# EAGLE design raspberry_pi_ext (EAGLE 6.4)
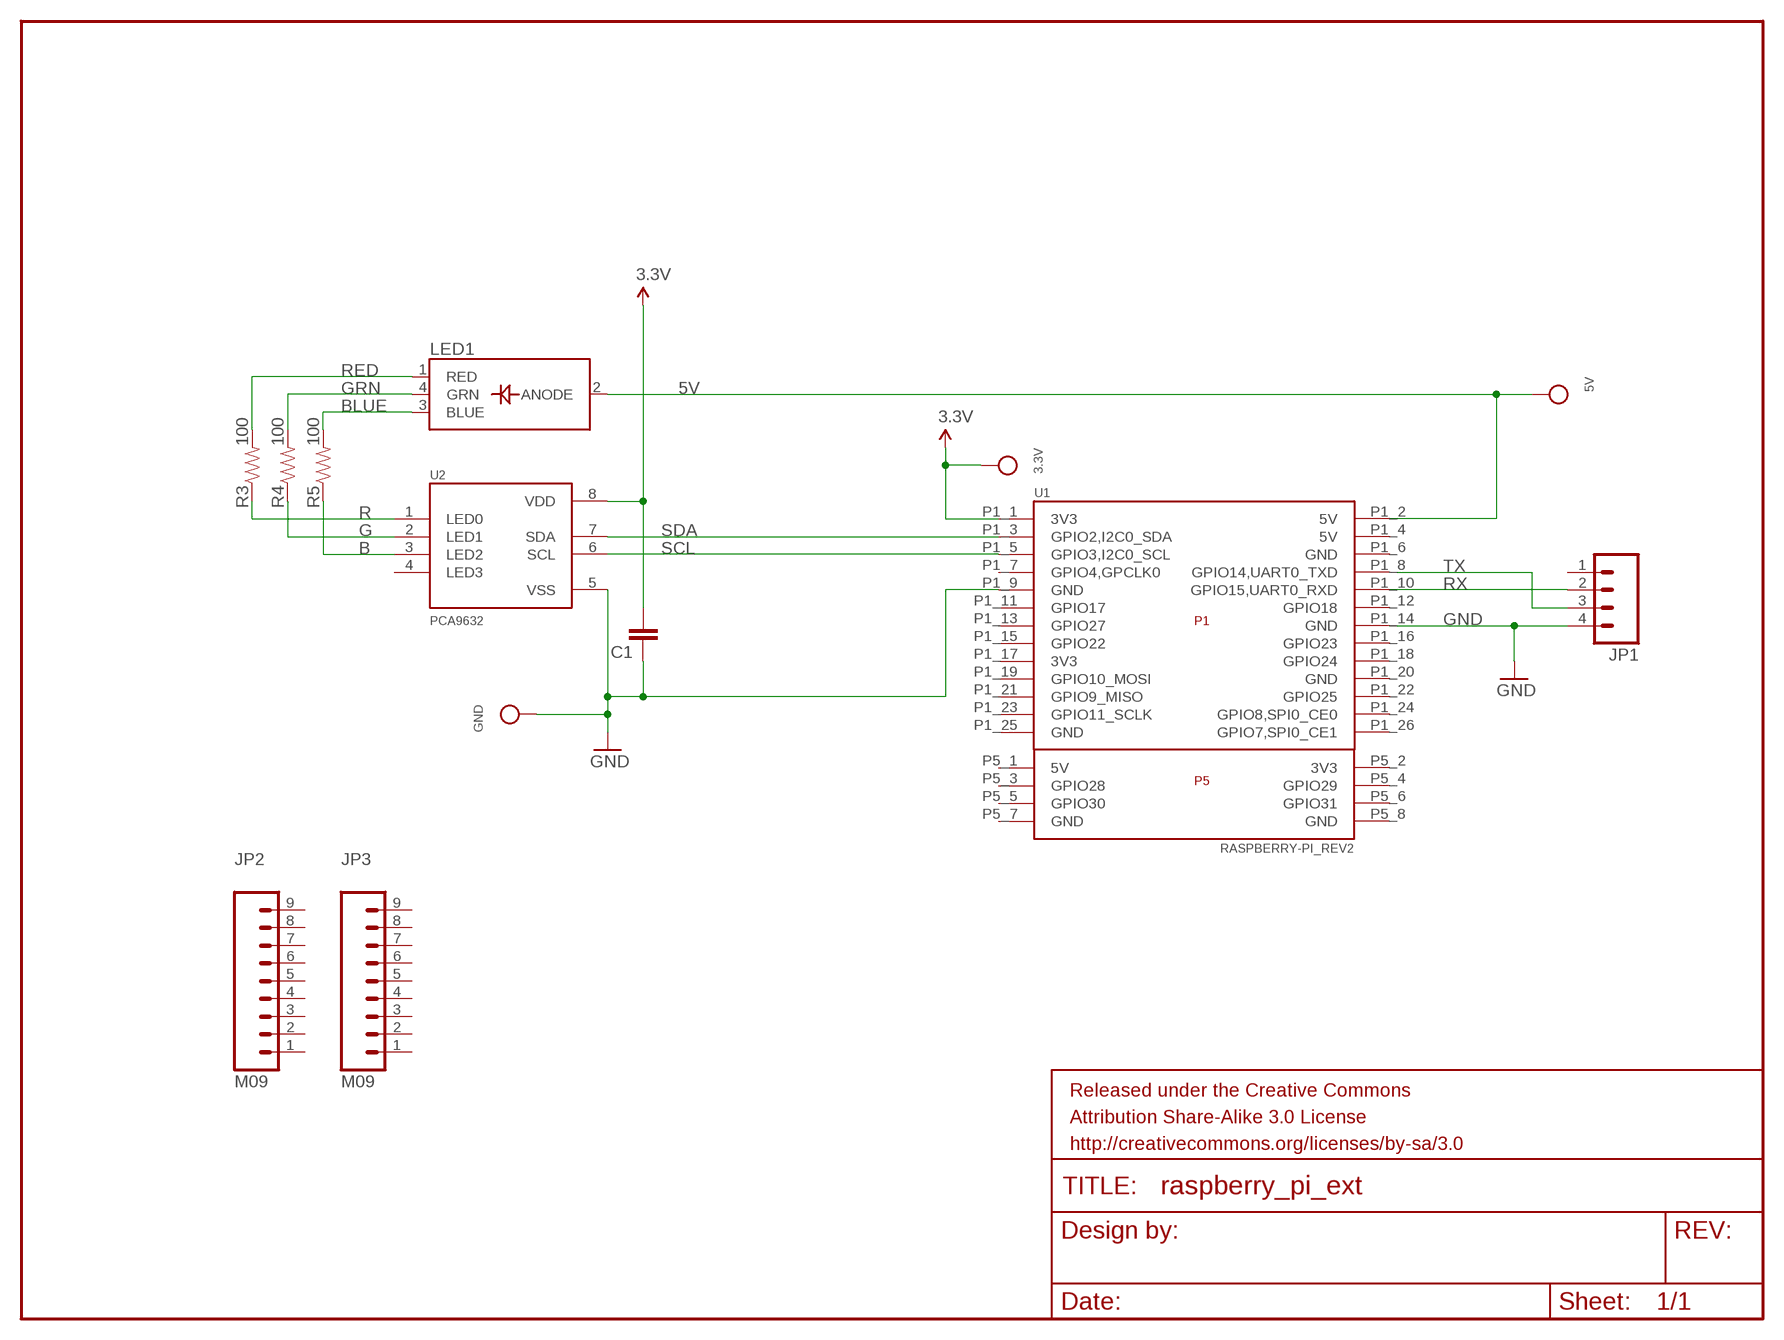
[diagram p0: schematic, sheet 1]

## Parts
3.3V  TESTPOINT0.1"  [1X01_ROUND]
5V  TESTPOINT0.1"  [1X01_ROUND]
C1  CAP0603-CAP  [0603-CAP]
FRAME1  FRAME-LETTER  [CREATIVE_COMMONS]
GND  TESTPOINT0.1"  [1X01_ROUND]
JP1  M04PTH  [1X04]
JP2  M09  [1X09]
JP3  M09  [1X09]
LED1  LED_RGB_PLCC4  [RGBLED_PLCC4]
R3  100  RESISTOR0603-RES  [0603-RES]
R4  100  RESISTOR0603-RES  [0603-RES]
R5  100  RESISTOR0603-RES  [0603-RES]
U1  RASPBERRY-PI_REV2  [RASPBERRY-PI_REV2]
U2  PCA9632  [TSSOP-8]

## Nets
3.3V: 3.3V.1 C1.2 U1.P1_1(3V3) U2.8(VDD)
5V: 5V.1 LED1.2(ANODE) U1.P1_2(5V)
B: R5.1 U2.3(LED2)
BLUE: LED1.3(BLUE) R5.2
G: R4.1 U2.2(LED1)
GND: C1.1 GND.1 JP1.4 U1.P1_9(GND) U1.P1_14(GND) U2.5(VSS)
GRN: LED1.4(GRN) R4.2
R: R3.1 U2.1(LED0)
RED: LED1.1(RED) R3.2
RX: JP1.2 U1.P1_10(GPIO15,UART0_RXD)
SCL: U1.P1_5(GPIO3,I2C0_SCL) U2.6(SCL)
SDA: U1.P1_3(GPIO2,I2C0_SDA) U2.7(SDA)
TX: JP1.3 U1.P1_8(GPIO14,UART0_TXD)
Unconnected: JP1.1 JP2.1 JP2.2 JP2.3 JP2.4 JP2.5 JP2.6 JP2.7 JP2.8 JP2.9 JP3.1 JP3.2 JP3.3 JP3.4 JP3.5 JP3.6 JP3.7 JP3.8 JP3.9 U1.P1_4(5V) U1.P1_6(GND) U1.P1_7(GPIO4,GPCLK0) U1.P1_11(GPIO17) U1.P1_12(GPIO18) U1.P1_13(GPIO27) U1.P1_15(GPIO22) U1.P1_16(GPIO23) U1.P1_17(3V3) U1.P1_18(GPIO24) U1.P1_19(GPIO10_MOSI) U1.P1_20(GND) U1.P1_21(GPIO9_MISO) U1.P1_22(GPIO25) U1.P1_23(GPIO11_SCLK) U1.P1_24(GPIO8,SPI0_CE0) U1.P1_25(GND) U1.P1_26(GPIO7,SPI0_CE1) U1.P5_1(5V) U1.P5_2(3V3) U1.P5_3(GPIO28) U1.P5_4(GPIO29) U1.P5_5(GPIO30) U1.P5_6(GPIO31) U1.P5_7(GND) U1.P5_8(GND) U2.4(LED3)

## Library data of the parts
3.3V 5V GND = microbuilder:TESTPOINT: Test Point; BOM: EXCLUDE
C1 = SparkFun-Capacitors:CAP: Capacitor
FRAME1 = SparkFun-Aesthetics:FRAME-LETTER: Schematic Frame
JP1 = SparkFun-Connectors:M04: Header 4 Standard 4-pin 0.1" header. Use with straight break away headers (SKU : PRT-00116), right angle break away headers (PRT-00553), swiss pins (PRT-00743), machine pins (PRT-00117), and female headers (PRT-00115). Molex polarized connector foot print use with SKU : PRT-08231 with associated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
JP2 JP3 = SparkFun-Connectors:M09: Header 9 Standard 9-pin 0.1" header. Use with straight break away headers (SKU : PRT-00116), right angle break away headers (PRT-00553), swiss pins (PRT-00743), machine pins (PRT-00117), and female headers (PRT-00115).
LED1 = microbuilder:LED_RGB_PLCC4: RGB LED - PLCC4 Cree 20mA Common Anode Digikey: CLV1A-FKB-CJ1M1F1BB7R4S3CT-ND Red: 2.6V Vf, 550mcd Green: 3.2V Vf, 850mcd Blue: 3.2V Vf, 320mcd
R3-R5 = SparkFun-Resistors:RESISTOR: Resistor
U1 = RaspberryPi:RASPBERRY-PI_REV2: Raspberry Pi Board Jacques Lagnel V1.0 (beta) 2012 Mateusz Bawaj V1.1 (beta) 2012 Board dimension: Forum 3D model The GPIO Connector (P1): http://elinux.org/RPi_Low-level_peripherals The GPIO Connector (P5): http://www.raspberrypi-spy.co.uk/2012/09/raspberry-pi-p5-header/
U2 = jetperch:PCA9632

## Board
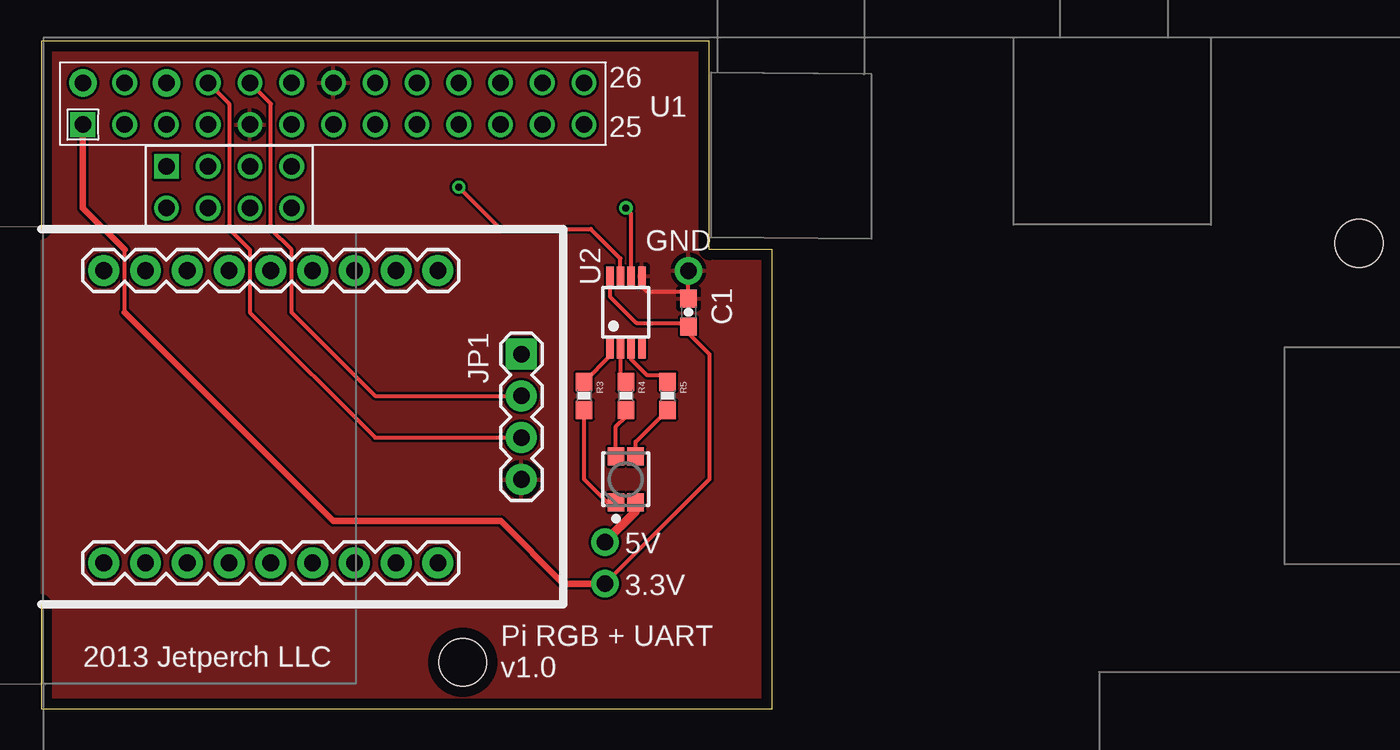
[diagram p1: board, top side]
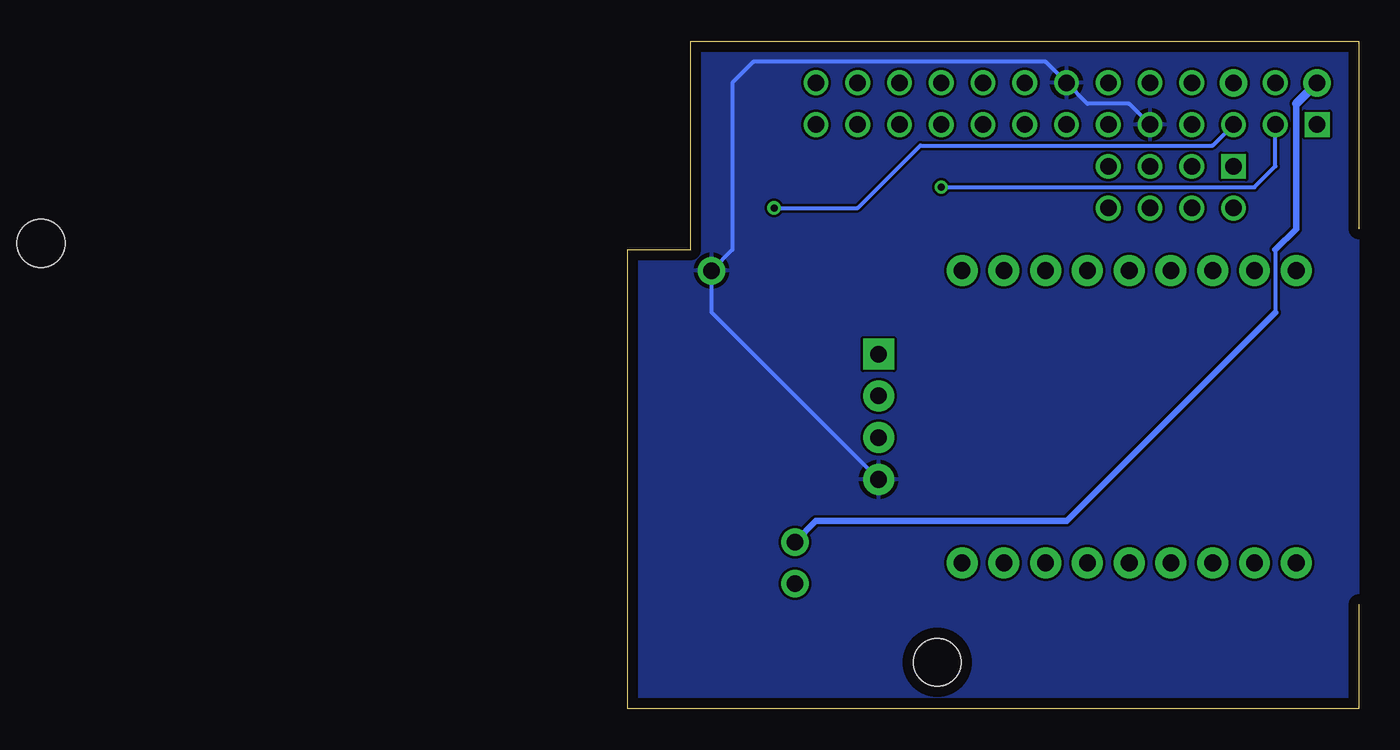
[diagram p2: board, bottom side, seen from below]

Size 44.45 x 40.64 mm. Coordinates in mm from the lower left corner, seen from the top.
Outline: 0,29.21 0,40.64 40.64,40.64 40.64,27.94 44.45,27.94 44.45,0 0,0 0,6.35
Copper layers (1*16): Top 0.035mm / dielectric 62mil / Bottom 0.035mm
Design rules "4pcb_33": minimum track width 6mil, minimum drill 15mil, track to track 6mil, track to pad 6mil, pad to pad 6mil, via to via 6mil, smd to smd 6mil, copper to edge 25mil, drill to drill 6mil, minimum pad ring 10mil, minimum via ring 8mil, stop-mask expansion 4mil, vias tented up to drill 25mil, thermal gap 10mil

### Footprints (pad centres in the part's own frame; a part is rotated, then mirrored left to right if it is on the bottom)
1X01_ROUND = drill 1 pad 1.676: 1 0,0
0603-CAP = smd 1.1 x 1: 1 -0.85,0; 2 0.85,0
1X04 = drill 1.016 pad 1.88 square: 1 0,0 | drill 1.016 pad 1.88: 2 2.54,0; 3 5.08,0; 4 7.62,0
1X09 = drill 1.016 pad 1.88: 1 0,0; 2 2.54,0; 3 5.08,0; 4 7.62,0; 5 10.16,0; 6 12.7,0; 7 15.24,0; 8 17.78,0; 9 20.32,0
RGBLED_PLCC4 = smd 1.1 x 1: 1 -1.4,0.6; 2 -1.4,-0.6; 3 1.4,-0.6; 4 1.4,0.6
0603-RES = smd 1.1 x 1: 1 -0.85,0; 2 0.85,0
RASPBERRY-PI_REV2 = drill 1 square: P1_1 -41.91,21.59; P5_1 -36.83,19.05 | drill 1 pad 1.676: P1_2 -41.91,24.13; P1_6 -36.83,24.13 | drill 1: P1_3 -39.37,21.59; P1_4 -39.37,24.13; P1_5 -36.83,21.59; P1_7 -34.29,21.59; P1_8 -34.29,24.13; P1_9 -31.75,21.59; P1_10 -31.75,24.13; P1_11 -29.21,21.59; P1_12 -29.21,24.13; P1_13 -26.67,21.59; P1_14 -26.67,24.13; P1_15 -24.13,21.59; P1_16 -24.13,24.13; P1_17 -21.59,21.59; P1_18 -21.59,24.13; P1_19 -19.05,21.59; P1_20 -19.05,24.13; P1_21 -16.51,21.59; P1_22 -16.51,24.13; P1_23 -13.97,21.59; P1_24 -13.97,24.13; P1_25 -11.43,21.59; P1_26 -11.43,24.13; P5_2 -36.83,16.51; P5_3 -34.29,19.05; P5_4 -34.29,16.51; P5_5 -31.75,19.05; P5_6 -31.75,16.51; P5_7 -29.21,19.05; P5_8 -29.21,16.51 | hole 2.9: 35.69,14.365; -18.81,-11.135
TSSOP-8 = smd 1.2 x 0.45: 1 -2.2,0.975; 2 -2.2,0.325; 3 -2.2,-0.325; 4 -2.2,-0.975; 5 2.2,-0.975; 6 2.2,-0.325; 7 2.2,0.325; 8 2.2,0.975

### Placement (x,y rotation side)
3.3V  34.29,7.62 0 top
5V  34.29,10.16 0 top
C1  39.37,24.13 270 top
FRAME1  not placed on the board
GND  39.37,26.67 0 top
JP1  29.21,21.59 270 top
JP2  3.81,8.89 0 top
JP3  3.81,26.67 0 top
LED1  35.56,13.97 90 top
R3  33.02,19.05 270 top
R4  35.56,19.05 270 top
R5  38.1,19.05 270 top
U1  44.45,13.97 0 top
U2  35.56,24.13 90 top

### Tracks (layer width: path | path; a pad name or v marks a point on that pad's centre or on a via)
3.3V
  Top 0.254: 3.3V.1 40.64,13.97 40.64,21.59 39.37,22.86 C1.2 39.16,23.5 36.2,23.5 34.59,25.11 U2.8 | 5.08,24.13 5.08,27.94
  Top 0.381: 3.3V.1 31.75,7.62 27.94,11.43 17.78,11.43 5.08,24.13 | 5.08,27.94 2.54,30.48 U1.P1_1
5V
  Top 0.254: LED1.2 36.16,12.03
  Top 0.508: 36.16,12.03 5V.1
  Bottom 0.254: 5.08,27.94 5.08,24.13
  Bottom 0.381: 3.81,36.83 3.81,29.21 5.08,27.94 | 5.08,24.13 17.78,11.43 33.02,11.43 5V.1
  Bottom 0.508: 3.81,36.83 U1.P1_2
B
  Top 0.254: U2.3 35.88,21.27 36.83,20.32 37.68,20.32 R5.1
BLUE
  Top 0.254: LED1.3 36.16,16.26 R5.2
G
  Top 0.254: U2.2 35.23,20.23 R4.1
GND
  Top 0.254: U2.5 36.53,25.7 36.83,25.4 38.95,25.4 C1.1 GND.1
  Bottom 0.254: JP1.4 39.37,24.13 GND.1 38.1,27.94 38.1,38.1 36.83,39.37 19.05,39.37 U1.P1_14 16.51,36.83 13.97,36.83 U1.P1_9
  pour Bottom: 0,0 44.45,0 44.45,27.94 40.64,27.94 40.64,40.64 0,40.64
  pour Top: 0,0 44.45,0 44.45,27.94 40.64,27.94 40.64,40.64 0,40.64
GRN
  Top 0.254: R4.2 35.56,17.78 34.92,17.14 34.92,15.4 LED1.4
R
  Top 0.254: U2.1 34.59,21.46 R3.1
RED
  Top 0.254: LED1.1 34.42,12.57 33.02,13.97 R3.2
RX
  Top 0.254: U1.P1_10 13.97,36.83 13.97,29.21 15.24,27.94 15.24,24.13 20.32,19.05 JP1.2
SCL  (via drill 0.41)
  Top 0.254: U2.6 35.88,30.16 v35.56,30.48
  Bottom 0.254: v35.56,30.48 30.48,30.48 26.67,34.29 8.89,34.29 U1.P1_5
SDA  (via drill 0.41)
  Top 0.254: U2.7 35.23,27.41 33.44,29.21 27.94,29.21 v25.4,31.75
  Bottom 0.254: v25.4,31.75 6.35,31.75 5.08,33.02 U1.P1_3
TX
  Top 0.254: U1.P1_8 11.43,36.83 11.43,29.21 12.7,27.94 12.7,24.13 20.32,16.51 JP1.3

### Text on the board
tNames: Pi RGB + UART | 2013 Jetperch LLC | v1.0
